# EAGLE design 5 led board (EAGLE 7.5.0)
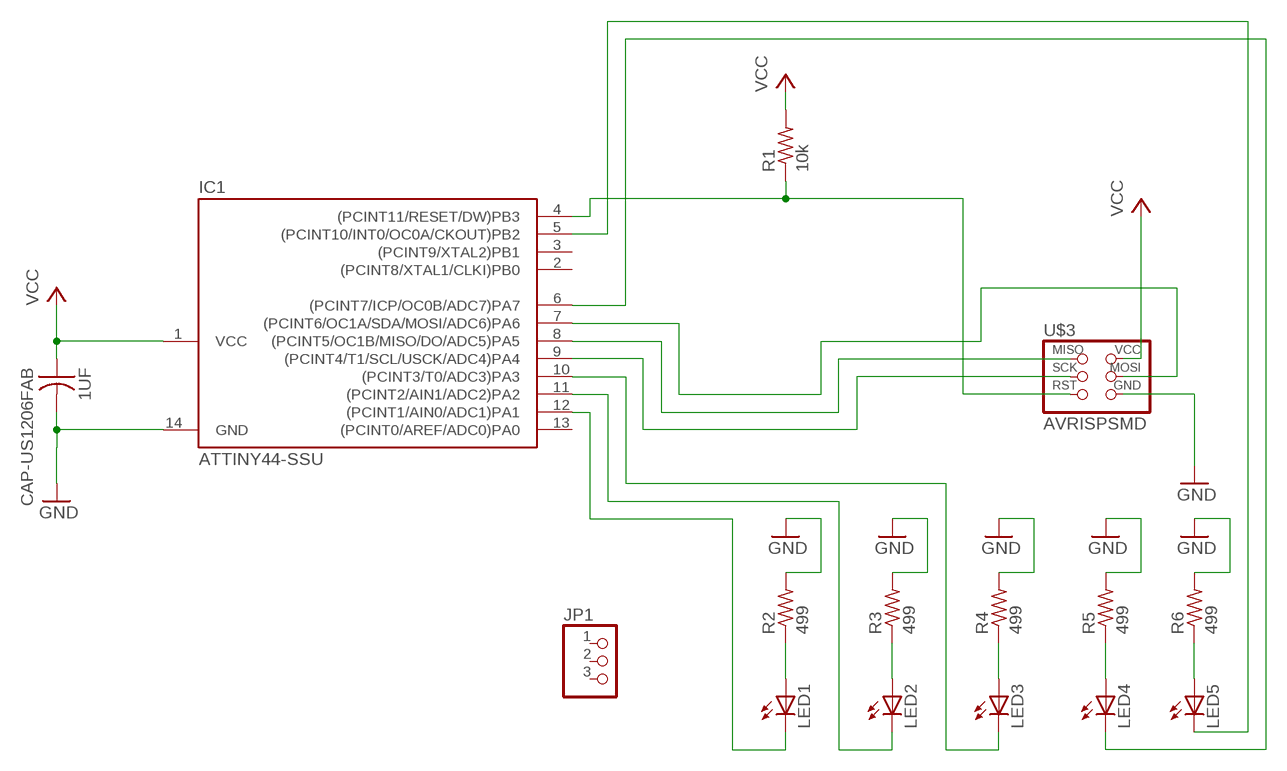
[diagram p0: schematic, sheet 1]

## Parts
1UF  CAP-US1206FAB  [C1206FAB]
IC1  ATTINY44-SSU  [SOIC14]
JP1  PINHD-1X3  [1X03]
LED1  LEDSML1206  [SML1206]
LED2  LEDSML1206  [SML1206]
LED3  LEDSML1206  [SML1206]
LED4  LEDSML1206  [SML1206]
LED5  LEDSML1206  [SML1206]
R1  10k  RES-US1206FAB  [R1206FAB]
R2  499  RES-US1206FAB  [R1206FAB]
R3  499  RES-US1206FAB  [R1206FAB]
R4  499  RES-US1206FAB  [R1206FAB]
R5  499  RES-US1206FAB  [R1206FAB]
R6  499  RES-US1206FAB  [R1206FAB]
U$3  AVRISPSMD  [2X03SMD]

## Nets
GND: 1UF.2 IC1.14(GND) R2.2 R3.2 R4.2 R5.2 R6.2 U$3.6(GND)
N$1: LED1.A R2.1
N$3: LED2.A R3.1
N$4: IC1.8((PCINT5/OC1B/MISO/DO/ADC5)PA5) U$3.1(MISO)
N$5: IC1.7((PCINT6/OC1A/SDA/MOSI/ADC6)PA6) U$3.4(MOSI)
N$6: IC1.10((PCINT3/T0/ADC3)PA3) LED3.C
N$8: LED3.A R4.1
N$10: LED4.A R5.1
N$11: IC1.11((PCINT2/AIN1/ADC2)PA2) LED2.C
N$12: IC1.9((PCINT4/T1/SCL/USCK/ADC4)PA4) U$3.3(SCK)
N$13: IC1.12((PCINT1/AIN0/ADC1)PA1) LED1.C
N$15: LED5.A R6.1
N$17: IC1.4((PCINT11/RESET/DW)PB3) R1.1 U$3.5(RST)
N$18: IC1.6((PCINT7/ICP/OC0B/ADC7)PA7) LED4.C
N$19: IC1.5((PCINT10/INT0/OC0A/CKOUT)PB2) LED5.C
VCC: 1UF.1 IC1.1(VCC) R1.2 U$3.2(VCC)
Unconnected: IC1.2((PCINT8/XTAL1/CLKI)PB0) IC1.3((PCINT9/XTAL2)PB1) IC1.13((PCINT0/AREF/ADC0)PA0) JP1.1 JP1.2 JP1.3

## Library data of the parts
1UF = fab:CAP-US
IC1 = fab:ATTINY44
JP1 = pinhead:PINHD-1X3: PIN HEADER
LED1-LED5 = led:LED: LED
R1-R6 = fab:RES-US: Resistor (US Symbol)
U$3 = fab:AVRISP

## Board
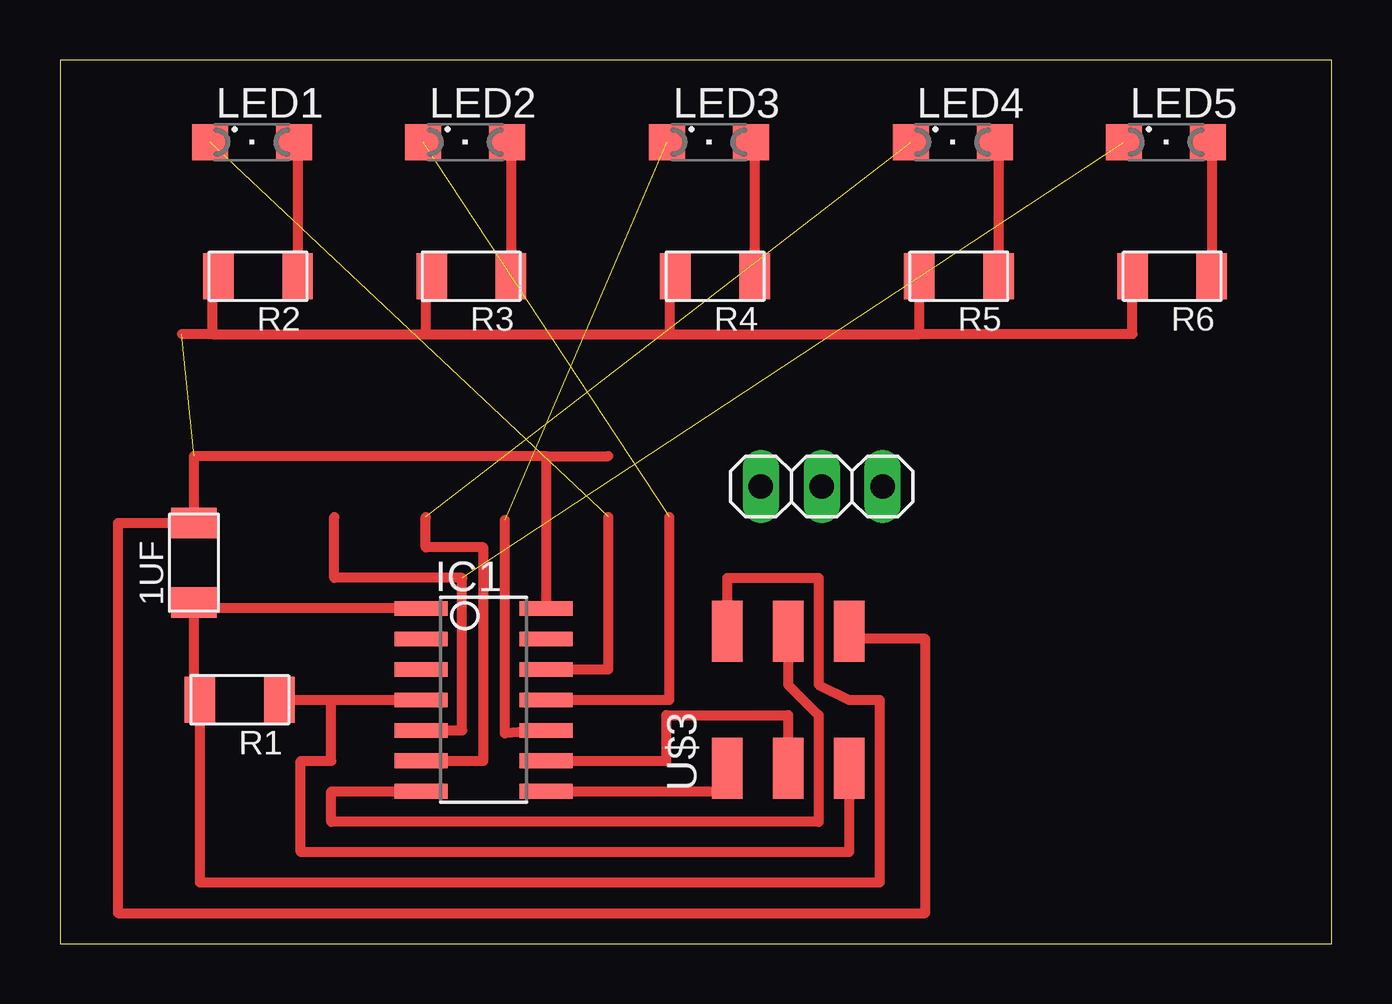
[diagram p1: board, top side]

Size 53.01 x 36.82 mm. Coordinates in mm from the lower left corner, seen from the top.
Outline: 0,0 53.01,0 53.01,36.82 0,36.82 0,0
Copper layers (1*16): Top 0.035mm / dielectric 1.5mm / Bottom 0.035mm
Design rules "default": minimum track width 10mil, minimum drill 24mil, track to track 8mil, track to pad 8mil, pad to pad 8mil, via to via 8mil, smd to smd 8mil, copper to edge 40mil, drill to drill 8mil, minimum pad ring 10mil, minimum via ring 8mil, stop-mask expansion 4mil, vias tented up to drill 0mil, thermal gap 10mil

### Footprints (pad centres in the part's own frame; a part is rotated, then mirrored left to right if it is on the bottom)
C1206FAB = smd 1.27 x 1.905: 1 -1.651,0; 2 1.651,0
SOIC14 = smd 0.61 x 2.21: 1 -3.81,-2.603; 2 -2.54,-2.603; 3 -1.27,-2.603; 4 0,-2.603; 5 1.27,-2.603; 6 2.54,-2.603; 7 3.81,-2.603; 8 3.81,2.603; 9 2.54,2.603; 10 1.27,2.603; 11 0,2.603; 12 -1.27,2.603; 13 -2.54,2.603; 14 -3.81,2.603
1X03 = drill 1.016 long: 1 -2.54,0; 2 0,0; 3 2.54,0
SML1206 = smd 1.5 x 1.5: A 1.75,0; C -1.75,0
R1206FAB = smd 1.27 x 1.905: 1 -1.651,0; 2 1.651,0
2X03SMD = smd 2.54 x 1.27: 1 -2.857,2.54; 2 2.857,2.54; 3 -2.857,0; 4 2.857,0; 5 -2.857,-2.54; 6 2.857,-2.54

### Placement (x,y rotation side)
1UF  5.59,15.88 90 top
IC1  17.65,10.16 270 top
JP1  31.75,19.05 0 top
LED1  8,33.4 0 top
LED2  16.89,33.4 0 top
LED3  27.05,33.4 0 top
LED4  37.21,33.4 0 top
LED5  46.1,33.4 0 top
R1  7.49,10.16 180 top
R2  8.26,27.81 180 top
R3  17.14,27.81 180 top
R4  27.3,27.81 180 top
R5  37.46,27.81 180 top
R6  46.35,27.81 180 top
U$3  30.35,10.16 90 top

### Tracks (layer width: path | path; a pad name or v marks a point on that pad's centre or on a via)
GND  (1 unrouted)
  Top 0.406: U$3.6 32.89,12.7 36.07,12.7 36.07,1.27 2.41,1.27 2.41,17.53 1UF.2 5.59,20.32 20.26,20.32 | 20.83,13.97 IC1.14 20.26,20.32 | 35.81,25.4 44.7,25.4 R6.2 | 35.81,25.4 R5.2 | R4.2 25.4,27.81 25.4,25.4 | 25.4,25.4 35.81,25.4 | R3.2 15.24,27.81 15.24,25.4 | 15.24,25.4 25.4,25.4 | R2.2 6.35,27.81 6.35,25.4 | 6.35,25.4 15.24,25.4 | 6.35,25.4 5.08,25.4 | 20.26,20.32 22.86,20.32
N$1
  Top 0.406: LED1.A 9.91,33.4 R2.1
N$3
  Top 0.406: LED2.A 18.8,33.4 R3.1
N$4
  Top 0.406: IC1.8 27.81,6.35 U$3.1
N$5
  Top 0.406: U$3.4 30.35,10.79 31.62,9.53 31.62,5.08 11.3,5.08 11.3,6.35 IC1.7
N$6  (1 unrouted)
  Top 0.406: IC1.10 18.54,8.76 18.54,17.65
N$8
  Top 0.406: LED3.A 28.96,33.4 R4.1
N$10
  Top 0.406: LED4.A 39.12,33.4 R5.1
N$11  (1 unrouted)
  Top 0.406: IC1.11 25.4,10.16 25.4,17.78
N$12
  Top 0.406: IC1.9 25.27,7.62 25.27,9.53 30.35,9.53 U$3.3
N$13  (1 unrouted)
  Top 0.406: IC1.12 22.86,11.43 22.86,17.78
N$15
  Top 0.406: LED5.A 48.01,33.4 R6.1
N$17
  Top 0.406: R1.1 11.3,10.16 | 11.3,10.16 IC1.4 | U$3.5 32.89,3.81 10.03,3.81 10.03,7.62 11.3,7.62 11.3,10.16
N$18  (1 unrouted)
  Top 0.406: IC1.6 17.65,7.62 17.65,16.51 15.24,16.51 15.24,17.78
N$19  (1 unrouted)
  Top 0.406: IC1.5 16.76,8.89 16.76,15.24 11.43,15.24 11.43,17.78
VCC
  Top 0.406: IC1.1 5.59,13.97 1UF.1 5.59,10.16 R1.2 5.84,2.54 34.16,2.54 34.16,10.16 32.89,10.16 31.62,10.79 31.62,15.24 27.81,15.24 U$3.2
